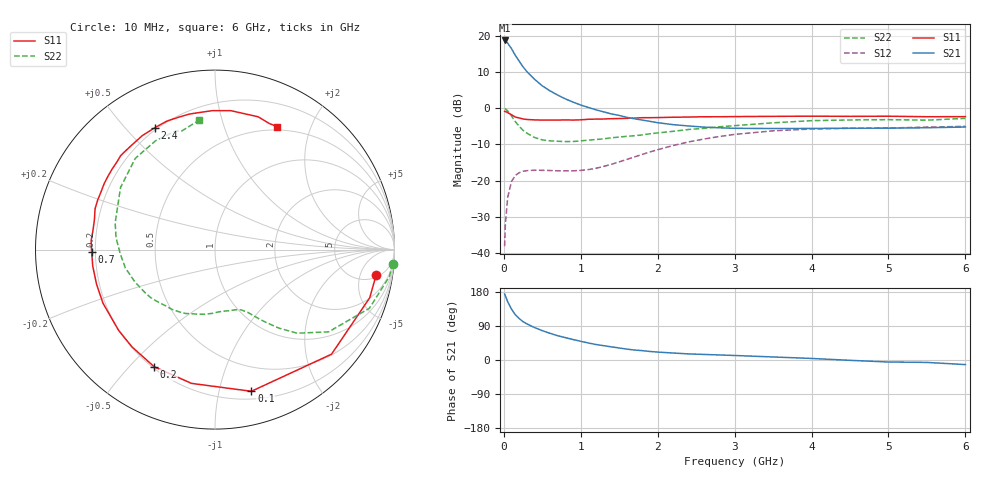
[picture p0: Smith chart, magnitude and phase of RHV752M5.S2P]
! SIEMENS Small Signal Semiconductors
! BFR106
! Si NPN RF Bipolar Junction Transistor in SOT23
! VCE = 0.75 V  IC = 2.5 mA
! Common Emitter S-Parameters:  August  1996
# GHz  S  MA  R  50
!  f  S11  S21  S12  S22
! GHz  MAG  ANG  MAG  ANG  MAG  ANG  MAG  ANG
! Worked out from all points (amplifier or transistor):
!   36 points, 10 MHz to 6 GHz, reference 50 ohm
!   highest |S21| = 18.8 dB at 10 MHz (marker M1)
!   |S21| within 3 dB of that: start of sweep to 119.2 MHz
!   unconditionally stable (mu >= 1): 712.3 MHz to end of sweep
!   at 250 MHz: K = 0.38, MSG = 14.4 dB, |S12| = -17.4 dB
!   at 1.4 GHz: K = 1.33, MAG = 3.5 dB, |S12| = -15.5 dB
!   at 6 GHz: K = 1.03, MAG = -1.1 dB, |S12| = -5.0 dB
!   S11 on the Smith chart (normalised r, x): 10 MHz: 6, -9; 100 MHz: 0.27, -1.25; 200 MHz: 0.21, -0.59; 700 MHz: 0.19, -0.01; 2.4 GHz: 0.19, +0.61; 6 GHz: 0.46, +1.53
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0.01  0.9089 -9.0  8.685 173.9  0.0124 86.1  0.992 -4.5
0.02  0.9028 -17.3  8.592 169.4  0.0251 82.2  0.9827 -8.8
0.05  0.8724 -41.9  7.987 153.6  0.0585 67.2  0.9204 -20.8
0.1  0.8151 -75.6  6.67 134.2  0.0977 50.7  0.7815 -35.9
0.15  0.7567 -100.0  5.396 119.2  0.1181 39.0  0.6531 -45.5
0.2  0.7356 -117.4  4.481 109.4  0.1286 32.2  0.5635 -50.9
0.25  0.7126 -130.4  3.745 101.1  0.1347 27.5  0.4949 -55.0
0.3  0.7007 -140.0  3.219 95.3  0.1374 24.6  0.4534 -57.8
0.4  0.6919 -154.4  2.517 85.6  0.1394 21.3  0.3948 -62.4
0.5  0.6876 -163.8  2.044 77.4  0.1388 20.2  0.366 -66.5
0.6  0.6873 -172.3  1.744 70.4  0.138 20.5  0.3544 -71.0
0.7  0.6875 -178.9  1.525 64.1  0.1366 22.0  0.3502 -76.1
0.9  0.6881 171.0  1.219 54.0  0.1367 27.6  0.3474 -86.5
1.1  0.7061 161.1  1.027 44.8  0.1422 35.0  0.363 -97.8
1.6  0.7276 142.2  0.751 28.7  0.1967 49.0  0.4105 -125.8
2.2  0.7532 122.5  0.595 18.4  0.3056 47.8  0.4808 -157.9
2.4  0.7574 116.2  0.57 16.1  0.3431 44.8  0.5098 -168.4
3  0.7686 100.7  0.529 11.9  0.4359 33.2  0.5759 165.0
3.5  0.7743 91.2  0.526 8.0  0.4884 23.3  0.6301 146.6
4.5  0.7746 77.1  0.531 -0.9  0.5288 6.2  0.6909 118.6
5.5  0.7652 66.9  0.539 -6.4  0.5494 -3.3  0.6864 105.6
6  0.767 63.2  0.551 -12.1  0.5635 -9.9  0.7263 97.0
